FUNCTION_BLOCK Example13_waituntilDI //4x3 flyways 1 xbot - waituntil DI, config DI as trigger
VAR_INPUT
	Execute : BOOL;
END_VAR
VAR_OUTPUT
	Done : BOOL;
END_VAR
VAR_IN_OUT
	PM_Controller : PMControllerType;	// the planar motor controller to use
END_VAR
VAR
	PMC_XYMotion1 : PMC_XYMotion;
	DI_ID_array22 : ARRAY[0..21] OF USINT;
	PMC_ConfigDI2Trigger1 : PMC_ConfigDI2Trigger;
	PMC_WaitUntilFBDI1 : PMC_WaitUntilFBDI;
	PMC_XYMotion2 : PMC_XYMotion;
	PMC_XYMotion3 : PMC_XYMotion;
	Delay1 : Delay;
	PMC_SendDigitalSignalToPMC1 : PMC_SendDigitalSignalToPMC;
	Delay2 : Delay;
	PMC_SendDigitalSignalToPMC2 : PMC_SendDigitalSignalToPMC;
END_VAR

//4x3 flyways 1 xbot - waituntil DI, config DI as trigger

//move xbot 1 to 60,60
PMC_XYMotion1(Execute := Execute,cmdLB := 1,XbotID := 1,Mode := 0,Type_ := 0,PosX := 0.06,PosY := 0.06,EndVel := 0,MaxVel := 1,MaxAcc := 10,PM_Controller := PM_Controller);

//set DI 1 as trigger source
DI_ID_array22[0] := 1;
PMC_ConfigDI2Trigger1(Execute := PMC_XYMotion1.Done,nDI := 1,DiID := DI_ID_array22,PM_Controller := PM_Controller);

//xbot 1 wait until DI1 rising edge
PMC_WaitUntilFBDI1(Execute := PMC_ConfigDI2Trigger1.Done,cmdLB := 3,XbotID := 1,TriggerDI := 1,TriggerType := 0,PM_Controller := PM_Controller);

//load xbot 1 move to 900,60
PMC_XYMotion2(Execute := PMC_WaitUntilFBDI1.Ack,cmdLB := 4,XbotID := 1,Mode := 0,Type_ := 0,PosX := 0.9,PosY := 0.06,EndVel := 0,MaxVel := 1,MaxAcc := 10,PM_Controller := PM_Controller);

//load xbot 1 move to 900,660
PMC_XYMotion3(Execute := PMC_XYMotion2.Ack,cmdLB := 5,XbotID := 1,Mode := 0,Type_ := 0,PosX := 0.9,PosY := 0.66,EndVel := 0,MaxVel := 1,MaxAcc := 10,PM_Controller := PM_Controller);

Delay1(Execute := PMC_XYMotion3.Ack,Cycles := 2000);

//set DI 1 to 0
PMC_SendDigitalSignalToPMC1(Enable := Delay1.Done,DoID := 1,Level := FALSE,PM_Controller := PM_Controller);

Delay2(Execute := PMC_SendDigitalSignalToPMC1.Valid,Cycles := 1);

//set DI 1 to 1
PMC_SendDigitalSignalToPMC2(Enable := Delay2.Done,DoID := 1,Level := TRUE,PM_Controller := PM_Controller);

Done := PMC_XYMotion3.Done;

END_FUNCTION_BLOCK
